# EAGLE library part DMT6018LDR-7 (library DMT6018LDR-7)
DIODES INC. - DMT6018LDR-7 - Dual MOSFET, N Channel, 60 V, 60 V, 8.8 A, 8.8 A, 0.013 ohm Source: Datasheet
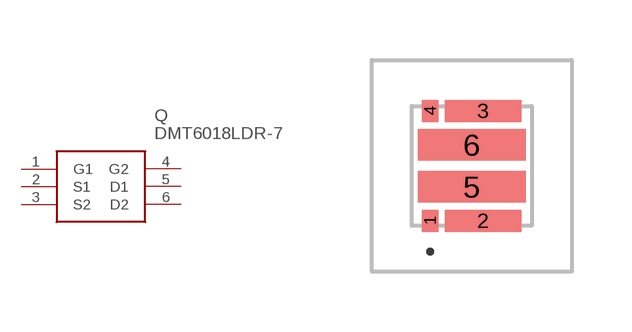
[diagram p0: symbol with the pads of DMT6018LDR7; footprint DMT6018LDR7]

Designator prefix Q

## DMT6018LDR-7 (Arrow_Part_Number: DMT6018LDR-7; Arrow_Price-Stock: https://www.arrow.com/en/products/dmt6018ldr-7/diodes-incorporated?utm_currency=USD&region=nac; Description: DIODES INC. - DMT6018LDR-7 - Dual MOSFET, N Channel, 60 V, 60 V, 8.8 A, 8.8 A, 0.013 ohm; Height: 0.85mm; Manufacturer_Name: Diodes Incorporated; Manufacturer_Part_Number: DMT6018LDR-7; Mouser_Part_Number: 621-DMT6018LDR-7; Mouser_Price-Stock: https://www.mouser.co.uk/ProductDetail/Diodes-Incorporated/DMT6018LDR-7?qs=4EhzHfbM1GhfDx1FS0oSLQ%3D%3D)  [DMT6018LDR7]
1  G1
2  S1
3  S2
4  G2
5  D1
6  D2

## Footprint DMT6018LDR7 (pad centres in mm)
V-DFN3030-8 (Type H)
smd 0.42 x 0.55: 1 -1.038,-1.375; 4 -1.038,1.375
smd 1.92 x 0.55: 2 0.287,-1.375; 3 0.287,1.375
smd 2.7 x 0.79: 5 0,-0.525; 6 0,0.525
